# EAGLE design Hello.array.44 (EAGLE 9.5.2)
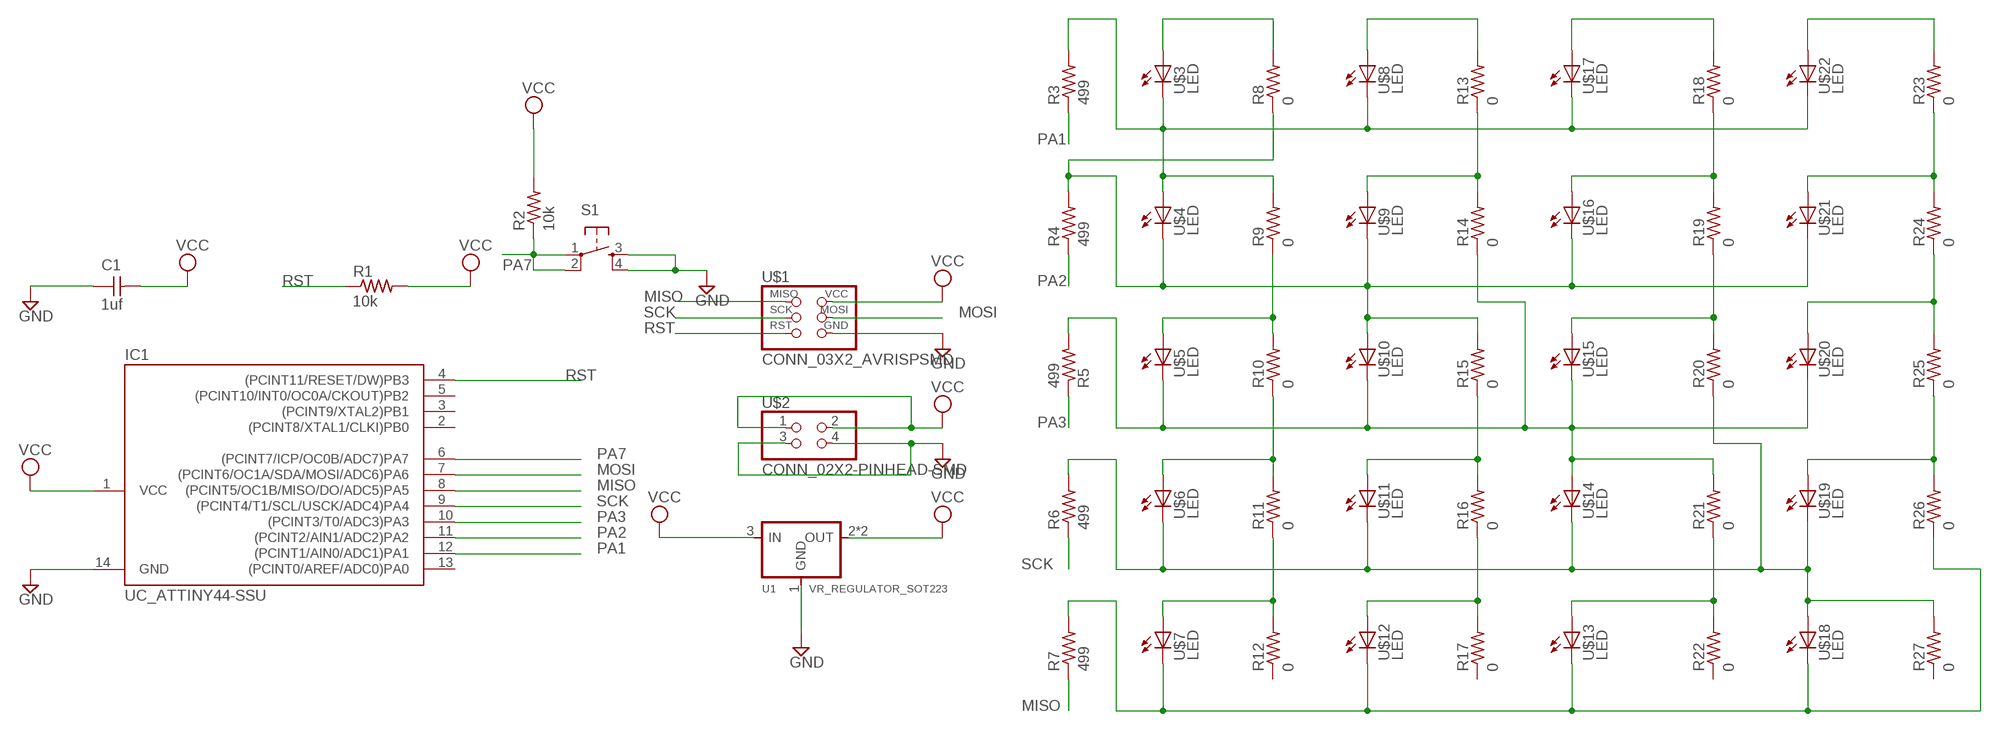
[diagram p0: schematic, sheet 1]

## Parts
C1  1uf  CAP_UNPOLARIZED  [C1206]
IC1  UC_ATTINY44-SSU  [SOIC14]
R1  10k  R1206  [R1206]
R2  10k  R1206  [R1206]
R3  499  R1206  [R1206]
R4  499  R1206  [R1206]
R5  499  R1206  [R1206]
R6  499  R1206  [R1206]
R7  499  R1206  [R1206]
R8  0  R1206  [R1206]
R9  0  R1206  [R1206]
R10  0  R1206  [R1206]
R11  0  R1206  [R1206]
R12  0  R1206  [R1206]
R13  0  R1206  [R1206]
R14  0  R1206  [R1206]
R15  0  R1206  [R1206]
R16  0  R1206  [R1206]
R17  0  R1206  [R1206]
R18  0  R1206  [R1206]
R19  0  R1206  [R1206]
R20  0  R1206  [R1206]
R21  0  R1206  [R1206]
R22  0  R1206  [R1206]
R23  0  R1206  [R1206]
R24  0  R1206  [R1206]
R25  0  R1206  [R1206]
R26  0  R1206  [R1206]
R27  0  R1206  [R1206]
S1  SW_SWITCH_TACTILE_6MM6MM_SWITCH  [6MM_SWITCH]
U1  VR_REGULATOR_SOT223  [SOT223]
U$1  CONN_03X2_AVRISPSMD  [2X03SMD]
U$2  CONN_02X2-PINHEAD-SMD  [2X02SMD]
U$3  LED  [LED1206]
U$4  LED  [LED1206]
U$5  LED  [LED1206]
U$6  LED  [LED1206]
U$7  LED  [LED1206]
U$8  LED  [LED1206]
U$9  LED  [LED1206]
U$10  LED  [LED1206]
U$11  LED  [LED1206]
U$12  LED  [LED1206]
U$13  LED  [LED1206]
U$14  LED  [LED1206]
U$15  LED  [LED1206]
U$16  LED  [LED1206]
U$17  LED  [LED1206]
U$18  LED  [LED1206]
U$19  LED  [LED1206]
U$20  LED  [LED1206]
U$21  LED  [LED1206]
U$22  LED  [LED1206]

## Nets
GND: C1.1 IC1.14(GND) S1.3(S) S1.4(S1) U1.1(GND) U$1.6(GND) U$2.3 U$2.4
MISO: IC1.8((PCINT5/OC1B/MISO/DO/ADC5)PA5) R7.1 U$1.1(MISO)
MOSI: IC1.7((PCINT6/OC1A/SDA/MOSI/ADC6)PA6) U$1.4(MOSI)
N$1: R13.2 U$8.1(A)
N$2: R3.2 R9.2 U$3.2(C) U$4.1(A) U$8.2(C) U$17.2(C) U$22.2(C)
N$3: R23.2 U$22.1(A)
N$4: R23.1 R24.2 U$21.1(A)
N$5: R24.1 R25.2 U$20.1(A)
N$6: R25.1 R26.2 U$19.1(A)
N$7: R8.2 U$3.1(A)
N$9: R13.1 R14.2 U$9.1(A)
N$10: R18.2 U$17.1(A)
N$11: R18.1 R19.2 U$16.1(A)
N$12: R4.2 R8.1 R15.2 U$4.2(C) U$9.2(C) U$10.1(A) U$16.2(C) U$21.2(C)
N$13: R15.1 R16.2 U$11.1(A)
N$15: R9.1 R10.2 U$5.1(A)
N$16: R6.2 R20.1 R27.2 U$6.2(C) U$11.2(C) U$14.2(C) U$18.1(A) U$19.2(C)
N$17: R5.2 R14.1 R21.2 U$5.2(C) U$10.2(C) U$14.1(A) U$15.2(C) U$20.2(C)
N$19: R19.1 R20.2 U$15.1(A)
N$21: R21.1 R22.2 U$13.1(A)
N$22: R16.1 R17.2 U$12.1(A)
N$24: R10.1 R11.2 U$6.1(A)
N$26: R11.1 R12.2 U$7.1(A)
N$27: R7.2 R26.1 U$7.2(C) U$12.2(C) U$13.2(C) U$18.2(C)
PA1: IC1.12((PCINT1/AIN0/ADC1)PA1) R3.1
PA2: IC1.11((PCINT2/AIN1/ADC2)PA2) R4.1
PA3: IC1.10((PCINT3/T0/ADC3)PA3) R5.1
PA7: IC1.6((PCINT7/ICP/OC0B/ADC7)PA7) R2.1 S1.1(P) S1.2(P1)
RST: IC1.4((PCINT11/RESET/DW)PB3) R1.1 U$1.5(RST)
SCK: IC1.9((PCINT4/T1/SCL/USCK/ADC4)PA4) R6.1 U$1.3(SCK)
VCC: C1.2 IC1.1(VCC) R1.2 R2.2 U1.2(OUT) U1.3(IN) U1.4(OUT) U$1.2(VCC) U$2.1 U$2.2
Unconnected: IC1.2((PCINT8/XTAL1/CLKI)PB0) IC1.3((PCINT9/XTAL2)PB1) IC1.5((PCINT10/INT0/OC0A/CKOUT)PB2) IC1.13((PCINT0/AREF/ADC0)PA0) R12.1 R17.1 R22.1 R27.1

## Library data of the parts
C1 = fab:CAP_UNPOLARIZED
IC1 = fab:UC_ATTINY44
R1-R27 = fab:R: Resistor (US Symbol)
S1 = fab:SW_SWITCH_TACTILE_6MM: OMRON SWITCH
U1 = fab:VR_REGULATOR_SOT223
U$1 = fab:CONN_03X2_AVRISP
U$2 = fab:CONN_02X2-PINHEAD-SMD
U$3-U$22 = fab:LED: LED

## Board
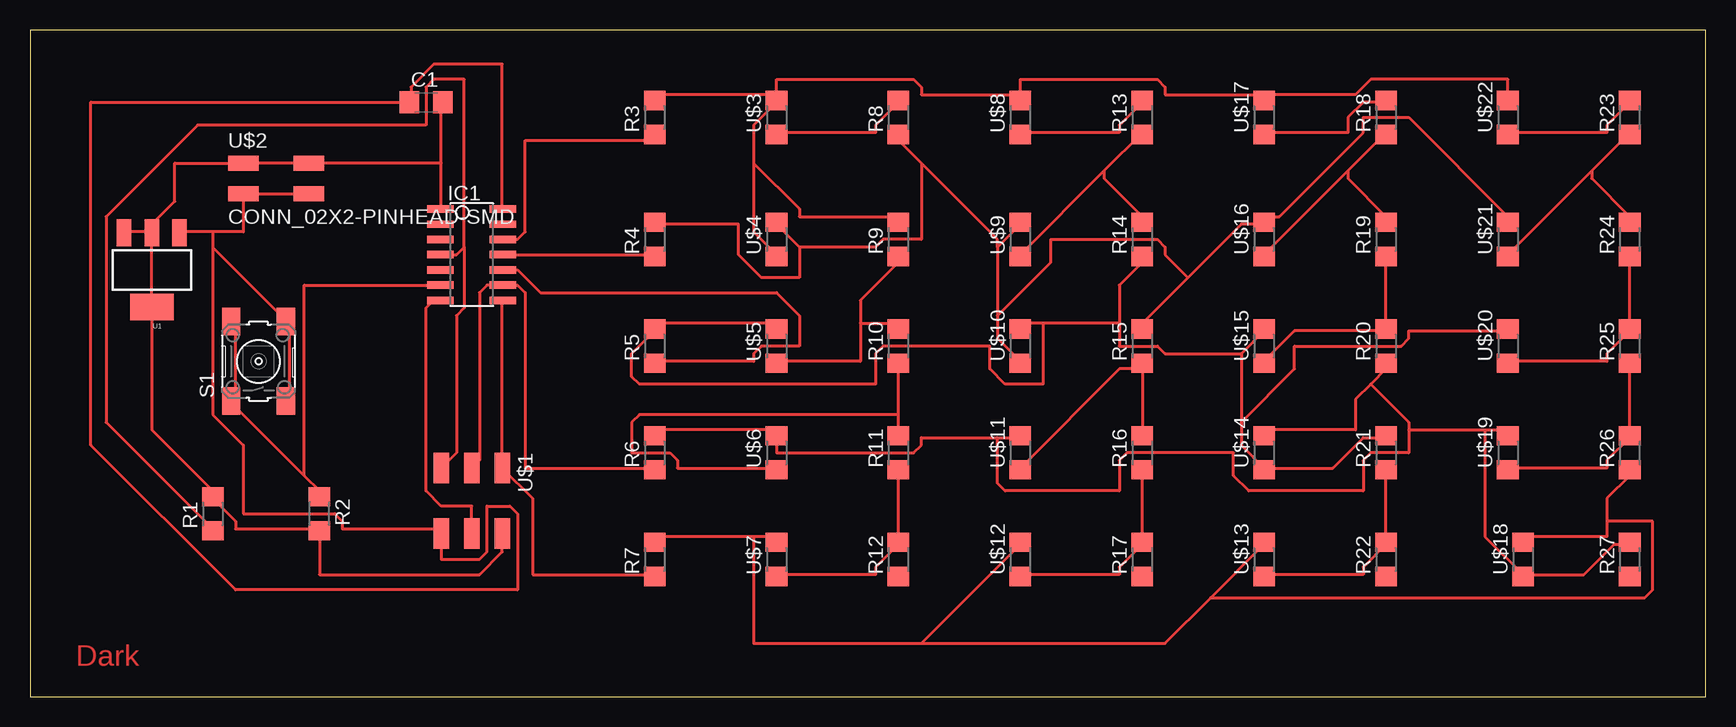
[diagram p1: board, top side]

Size 139.68 x 55.55 mm. Coordinates in mm from the lower left corner, seen from the top.
Outline: 0,0 139.68,0 139.68,55.55 0,55.55 0,0
Copper layers (1*16): Top 0.035mm / dielectric 1.5mm / Bottom 0.035mm
Design rules "fab": minimum track width 10mil, minimum drill 32mil, track to track 16mil, track to pad 16mil, pad to pad 16mil, via to via 16mil, smd to smd 6mil, copper to edge 16mil, drill to drill 16mil, minimum pad ring 10mil, minimum via ring 8mil, stop-mask expansion 4mil, vias tented up to drill 0mil, thermal gap 16mil

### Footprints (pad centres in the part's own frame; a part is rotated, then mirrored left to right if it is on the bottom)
C1206 = smd 1.6 x 1.8: 1 -1.4,0; 2 1.4,0
SOIC14 = smd 0.61 x 2.21: 1 -3.81,-2.603; 2 -2.54,-2.603; 3 -1.27,-2.603; 4 0,-2.603; 5 1.27,-2.603; 6 2.54,-2.603; 7 3.81,-2.603; 8 3.81,2.603; 9 2.54,2.603; 10 1.27,2.603; 11 0,2.603; 12 -1.27,2.603; 13 -2.54,2.603; 14 -3.81,2.603
R1206 = smd 1.6 x 1.803: 1 -1.422,0; 2 1.422,0
6MM_SWITCH = smd 2.286 x 1.524: 1 -3.302,2.286; 2 3.302,2.286; 3 -3.302,-2.286; 4 3.302,-2.286
SOT223 = smd 1.219 x 2.235: 1 -2.311,-3.099; 2 0,-3.099; 3 2.311,-3.099 | smd 3.6 x 2.2: 4 0,3.099
2X03SMD = smd 2.54 x 1.27: 1 -2.54,2.54; 2 2.92,2.54; 3 -2.54,0; 4 2.92,0; 5 -2.54,-2.54; 6 2.92,-2.54
2X02SMD = smd 2.54 x 1.27: 1 -2.54,1.27; 2 2.92,1.27; 3 -2.54,-1.27; 4 2.92,-1.27
LED1206 = smd 1.6 x 1.803: 1 -1.422,0; 2 1.422,0

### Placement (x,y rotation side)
C1  33.02,49.53 0 top
IC1  36.83,36.83 270 top
R1  15.24,15.24 90 top
R2  24.13,15.24 270 top
R3  52.07,48.26 90 top
R4  52.07,38.1 90 top
R5  52.07,29.21 90 top
R6  52.07,20.32 90 top
R7  52.07,11.43 90 top
R8  72.39,48.26 90 top
R9  72.39,38.1 90 top
R10  72.39,29.21 90 top
R11  72.39,20.32 90 top
R12  72.39,11.43 90 top
R13  92.71,48.26 90 top
R14  92.71,38.1 90 top
R15  92.71,29.21 90 top
R16  92.71,20.32 90 top
R17  92.71,11.43 90 top
R18  113.03,48.26 90 top
R19  113.03,38.1 90 top
R20  113.03,29.21 90 top
R21  113.03,20.32 90 top
R22  113.03,11.43 90 top
R23  133.35,48.26 90 top
R24  133.35,38.1 90 top
R25  133.35,29.21 90 top
R26  133.35,20.32 90 top
R27  133.35,11.43 90 top
S1  19.05,27.94 90 top
U1  10.16,35.56 180 top
U$1  36.83,16.51 270 top
U$2  20.32,43.18 0 top
U$3  62.23,48.26 90 top
U$4  62.23,38.1 90 top
U$5  62.23,29.21 90 top
U$6  62.23,20.32 90 top
U$7  62.23,11.43 90 top
U$8  82.55,48.26 90 top
U$9  82.55,38.1 90 top
U$10  82.55,29.21 90 top
U$11  82.55,20.32 90 top
U$12  82.55,11.43 90 top
U$13  102.87,11.43 90 top
U$14  102.87,20.32 90 top
U$15  102.87,29.21 90 top
U$16  102.87,38.1 90 top
U$17  102.87,48.26 90 top
U$18  124.46,11.43 90 top
U$19  123.19,20.32 90 top
U$20  123.19,29.21 90 top
U$21  123.19,38.1 90 top
U$22  123.19,48.26 90 top

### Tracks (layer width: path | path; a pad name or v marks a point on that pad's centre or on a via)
GND
  Top 0.254: IC1.14 39.37,40.64 39.37,52.7 33.66,52.7 31.75,50.8 31.75,49.53 C1.1 5.08,49.53 5.08,20.95 17.14,8.89 40.64,8.89 40.64,15.24 40,15.87 38.1,15.87 38.1,12.06 37.46,11.43 34.29,11.43 U$1.6 34.29,13.97 26.03,13.97 26.03,14.6 25.4,15.24 17.78,15.24 17.78,20.95 15.24,23.49 15.24,37.47 | S1.3 21.59,24.77 21.59,31.12 S1.4 20.95,31.75 15.24,37.47 | 15.24,38.73 17.78,38.73 U$2.3 U$2.4 | 15.24,38.73 12.7,38.73 U1.1 | 15.24,38.73 15.24,37.47
MISO
  Top 0.254: R7.1 52.07,10.16 41.91,10.16 41.91,16.51 U$1.1 39.37,33.02 IC1.8
MOSI
  Top 0.254: U$1.4 36.83,15.87 34.29,15.87 33.02,17.15 33.02,32.39 33.66,33.02 IC1.7
N$1
  Top 0.254: U$8.1 82.55,46.99 90.81,46.99 90.81,47.62 92.71,49.53 R13.2
N$2
  Top 0.254: 102.87,50.16 110.49,50.16 111.76,51.44 123.19,51.44 U$22.2 | 60.32,44.45 60.32,47.62 62.23,49.53 U$3.2 62.23,50.16 | 60.32,44.45 60.32,38.73 62.23,36.83 U$4.1 | 62.23,50.16 52.07,50.16 R3.2 | 60.32,44.45 64.14,40.64 64.14,40.01 72.39,40.01 R9.2 | 82.55,50.16 74.3,50.16 74.3,50.8 73.66,51.44 62.23,51.44 62.23,50.16 | 102.87,50.16 94.62,50.16 94.62,50.8 93.98,51.44 82.55,51.44 82.55,50.16 | 102.87,50.16 U$17.2 | 82.55,50.16 U$8.2
N$3
  Top 0.254: U$22.1 123.19,46.99 131.44,46.99 131.44,47.62 133.35,49.53 R23.2
N$4
  Top 0.254: 130.17,43.82 133.35,46.99 R23.1 | 130.17,43.82 123.19,36.83 U$21.1 | 130.17,43.82 130.17,43.18 133.35,40.01 R24.2
N$5
  Top 0.254: U$20.1 123.19,27.94 131.44,27.94 131.44,28.58 133.35,30.48 R25.2 R24.1
N$6
  Top 0.254: U$19.1 123.19,19.05 131.44,19.05 131.44,19.69 133.35,21.59 R26.2 R25.1
N$7
  Top 0.254: U$3.1 62.23,46.99 70.48,46.99 70.48,47.62 72.39,49.53 R8.2
N$9
  Top 0.254: 89.54,43.82 92.71,46.99 R13.1 | 89.54,43.82 82.55,36.83 U$9.1 | 89.54,43.82 89.54,43.18 92.71,40.01 R14.2
N$10
  Top 0.254: U$17.1 102.87,46.99 109.86,46.99 109.86,48.26 111.12,49.53 113.03,49.53 R18.2
N$11
  Top 0.254: 109.86,43.82 113.03,46.99 R18.1 | 109.86,43.82 102.87,36.83 U$16.1 | 109.86,43.82 109.86,43.18 113.03,40.01 R19.2
N$12
  Top 0.254: 96.52,34.93 100.97,39.37 102.87,39.37 U$16.2 102.87,40.01 104.14,40.01 111.12,46.99 111.12,48.26 114.94,48.26 123.19,40.01 U$21.2 | 96.52,34.93 92.71,31.12 R15.2 | 64.14,37.47 64.14,34.93 60.96,34.93 59.05,36.83 59.05,39.37 52.07,39.37 R4.2 | 64.14,37.47 62.23,39.37 U$4.2 | 80.65,37.47 80.65,31.75 | 80.65,31.75 80.65,29.84 82.55,27.94 U$10.1 | 80.65,37.47 82.55,39.37 U$9.2 | 74.3,44.45 80.65,38.1 80.65,37.47 | 74.3,44.45 72.39,46.36 R8.1 | 64.14,37.47 70.48,37.47 71.12,38.1 74.3,38.1 74.3,44.45 | 96.52,34.93 94.62,36.83 94.62,37.47 93.98,38.1 85.09,38.1 85.09,36.2 80.65,31.75
N$13
  Top 0.254: 92.71,27.3 90.81,27.3 82.55,19.05 U$11.1 | 92.71,27.3 R16.2 | 92.71,27.3 R15.1
N$15
  Top 0.254: 69.22,31.12 69.22,33.02 72.39,36.2 R9.1 | 69.22,31.12 69.22,27.94 62.23,27.94 U$5.1 | 69.22,31.12 72.39,31.12 R10.2
N$16
  Top 0.254: R6.2 52.07,22.23 62.23,22.23 U$6.2 62.23,20.32 73.66,20.32 74.3,20.95 74.3,21.59 80.65,21.59 | 80.65,21.59 82.55,21.59 U$11.2 | 111.76,26.03 113.03,27.3 R20.1 | 111.76,26.03 110.49,24.77 110.49,22.23 102.87,22.23 U$14.2 | 114.94,22.23 121.29,22.23 | 121.29,22.23 123.19,22.23 U$19.2 | 114.94,22.23 114.94,22.86 111.76,26.03 | 124.46,10.16 121.29,13.33 121.29,22.23 | 124.46,10.16 129.54,10.16 132.08,12.7 133.35,12.7 R27.2 | 124.46,10.16 U$18.1 | 80.65,21.59 80.65,17.78 81.28,17.15 90.81,17.15 90.81,19.69 91.44,20.32 100.33,20.32 100.33,18.41 101.6,17.15 111.12,17.15 111.12,19.69 111.76,20.32 114.94,20.32 114.94,22.23
N$17
  Top 0.254: 102.87,19.05 100.97,20.95 100.97,22.86 | 100.97,28.58 100.97,22.86 | 100.97,28.58 102.87,30.48 U$15.2 | 102.87,19.05 108.59,19.05 111.12,21.59 113.03,21.59 R21.2 | 102.87,19.05 U$14.1 | 100.97,22.86 105.41,27.3 105.41,29.21 114.3,29.21 114.94,29.84 114.94,30.48 123.19,30.48 U$20.2 | U$5.2 62.23,31.12 52.07,31.12 R5.2 52.07,30.48 50.16,28.58 50.16,26.67 50.8,26.03 70.48,26.03 70.48,28.58 71.12,29.21 80.01,29.21 80.01,27.3 81.28,26.03 84.45,26.03 84.45,31.12 | 90.81,31.12 84.45,31.12 | 84.45,31.12 82.55,31.12 U$10.2 | 90.81,31.12 90.81,34.29 92.71,36.2 R14.1 | 100.97,28.58 94.62,28.58 93.98,29.21 90.81,29.21 90.81,31.12
N$19
  Top 0.254: U$15.1 102.87,27.94 105.41,30.48 113.03,30.48 R20.2 R19.1
N$21
  Top 0.254: U$13.1 102.87,10.16 111.12,10.16 111.12,10.79 113.03,12.7 R22.2 R21.1
N$22
  Top 0.254: U$12.1 82.55,10.16 90.81,10.16 90.81,10.79 92.71,12.7 R17.2 R16.1
N$24
  Top 0.254: 72.39,23.49 50.8,23.49 50.16,22.86 50.16,20.32 53.34,20.32 53.98,19.69 53.98,19.05 62.23,19.05 U$6.1 | R11.2 72.39,23.49 | 72.39,23.49 R10.1
N$26
  Top 0.254: U$7.1 62.23,10.16 70.48,10.16 70.48,10.79 72.39,12.7 R12.2 R11.1
N$27
  Top 0.254: 131.44,14.6 131.44,16.51 133.35,18.41 R26.1 | 131.44,14.6 131.44,13.33 124.46,13.33 U$18.2 | 60.32,13.33 62.23,13.33 U$7.2 | 60.32,13.33 52.07,13.33 R7.2 | 74.3,4.45 82.55,12.7 U$12.2 | 74.3,4.45 60.32,4.45 60.32,13.33 | 98.43,8.26 94.62,4.45 74.3,4.45 | 98.43,8.26 102.87,12.7 U$13.2 | 131.44,14.6 135.25,14.6 135.25,8.89 134.62,8.26 98.43,8.26
PA1
  Top 0.254: IC1.12 40.64,38.1 41.27,38.73 41.27,46.36 52.07,46.36 R3.1
PA2
  Top 0.254: IC1.11 52.07,36.83 R4.1
PA3
  Top 0.254: IC1.10 40.64,35.56 42.54,33.66 62.23,33.66 64.14,31.75 64.14,29.21 60.96,29.21 60.32,28.58 60.32,27.94 52.07,27.94 R5.1
PA7
  Top 0.254: 22.86,18.41 17.14,24.13 S1.1 17.14,24.77 17.14,31.12 S1.2 | 22.86,18.41 24.13,17.15 R2.1 | IC1.6 22.86,34.29 22.86,18.41
RST
  Top 0.254: 36.2,37.47 36.2,51.44 33.66,51.44 33.02,50.8 33.02,47.62 13.97,47.62 6.35,40.01 6.35,22.86 15.24,13.97 R1.1 | 36.2,37.47 35.56,36.83 IC1.4 | U$1.5 35.56,20.32 35.56,31.75 36.2,32.39 36.2,37.47
SCK
  Top 0.254: R6.1 52.07,19.05 41.27,19.05 41.27,33.66 40.64,34.29 IC1.9 38.1,34.29 37.46,33.66 37.46,19.69 U$1.3
VCC
  Top 0.254: 34.29,44.45 34.29,40.64 IC1.1 | 34.29,44.45 34.29,49.53 C1.2 | 34.29,44.45 U$2.2 U$2.1 12.06,44.45 12.06,41.27 10.16,39.37 10.16,38.73 | 10.16,38.73 8.26,38.73 U1.3 | U$1.2 39.37,12.06 37.46,10.16 24.13,10.16 R2.2 24.13,13.97 17.14,13.97 17.14,14.6 15.24,16.51 R1.2 15.24,17.15 10.16,22.23 U1.4 U1.2 10.16,38.73

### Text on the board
Top: Dark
